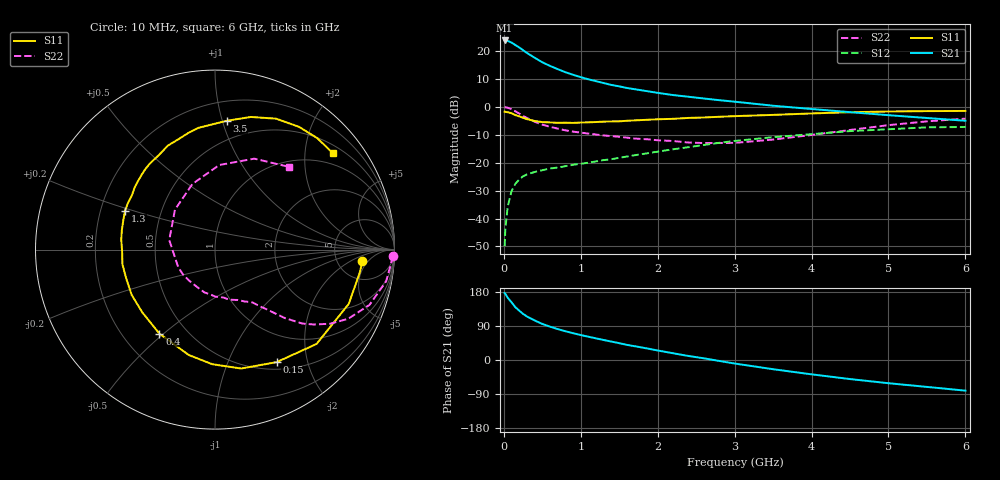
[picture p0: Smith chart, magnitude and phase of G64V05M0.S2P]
! SIEMENS Small Signal Semiconductors
! BFG193
! Si NPN RF Bipolar Junction Transistor in SOT223
! VCE = 4 V  IC = 5 mA
! Common Emitter S-Parameters:  August  1996
# GHz  S  MA  R  50
!  f  S11  S21  S12  S22
! GHz  MAG  ANG  MAG  ANG  MAG  ANG  MAG  ANG
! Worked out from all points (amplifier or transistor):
!   36 points, 10 MHz to 6 GHz, reference 50 ohm
!   highest |S21| = 23.8 dB at 10 MHz (marker M1)
!   |S21| within 3 dB of that: start of sweep to 224.8 MHz
!   unconditionally stable (mu >= 1): 1.1 GHz to 2.529 GHz
!   at 250 MHz: K = 0.34, MSG = 22.6 dB, |S12| = -24.9 dB
!   at 1.4 GHz: K = 1.08, MAG = 11.6 dB, |S12| = -18.7 dB
!   at 6 GHz: K = 0.87, MSG = 1.1 dB, |S12| = -7.2 dB
!   S11 on the Smith chart (normalised r, x): 10 MHz: 8.90, -3.58; 150 MHz: 0.59, -1.52; 400 MHz: 0.35, -0.48; 1.3 GHz: 0.31, +0.19; 3.5 GHz: 0.35, +1.03; 6 GHz: 0.69, +2.64
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0.01  0.8239 -4.5  15.55 176.8  0.0032 91.5  0.9912 -2.1
0.02  0.8165 -9.1  15.54 174.6  0.0065 87.0  0.9849 -4.2
0.05  0.8043 -22.1  15.28 164.4  0.0164 77.6  0.9697 -10.5
0.1  0.7724 -42.9  14.27 152.3  0.0311 70.1  0.9142 -19.7
0.15  0.7148 -61.3  12.87 139.3  0.042 60.0  0.8356 -27.5
0.2  0.6784 -77.6  11.66 130.2  0.0501 54.6  0.7625 -32.8
0.25  0.6387 -91.4  10.39 121.7  0.0571 49.6  0.6903 -37.2
0.3  0.6051 -104.0  9.302 114.9  0.0618 46.3  0.6365 -40.3
0.4  0.5613 -123.5  7.622 104.4  0.0683 41.9  0.5432 -44.5
0.5  0.5352 -139.2  6.318 95.2  0.0735 39.5  0.4817 -47.0
0.6  0.5285 -151.5  5.444 88.0  0.0788 38.5  0.4405 -49.1
0.7  0.5201 -162.2  4.765 81.6  0.0822 38.3  0.4089 -51.2
0.9  0.5177 -179.1  3.772 70.7  0.0919 38.5  0.3613 -54.6
1.1  0.5303 168.0  3.127 61.4  0.1003 39.0  0.3333 -60.2
1.3  0.546 156.7  2.675 52.7  0.1116 39.4  0.3084 -65.5
1.6  0.566 142.3  2.188 39.9  0.1292 38.6  0.2824 -76.4
2.2  0.6128 120.6  1.634 17.8  0.1743 33.8  0.2454 -104.2
2.8  0.6669 102.8  1.323 -2.5  0.2275 24.9  0.2264 -141.5
3.5  0.7206 84.8  1.052 -24.3  0.2875 10.1  0.2604 168.2
4.5  0.8049 65.0  0.807 -50.3  0.3694 -10.6  0.3867 109.0
5.5  0.8427 47.5  0.634 -71.0  0.4309 -36.6  0.5521 66.6
6  0.8485 39.3  0.566 -80.9  0.4376 -51.4  0.6172 48.4
